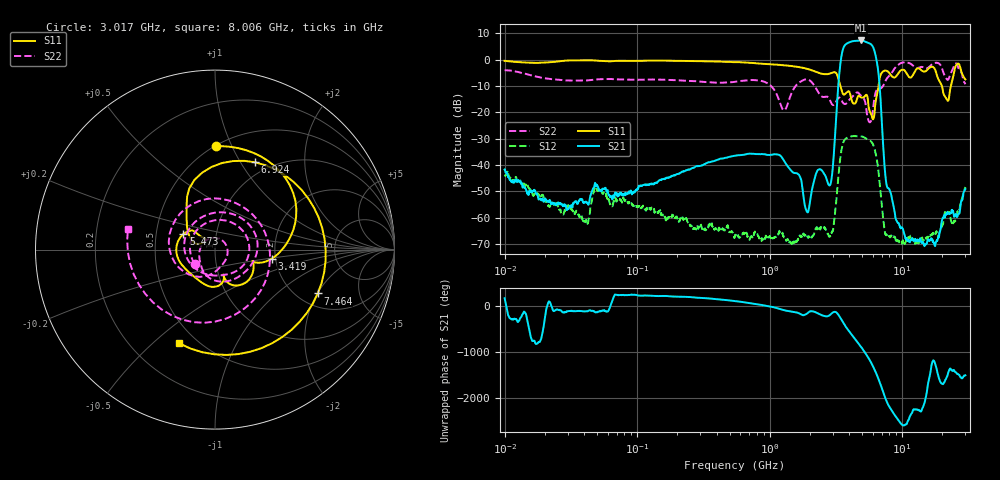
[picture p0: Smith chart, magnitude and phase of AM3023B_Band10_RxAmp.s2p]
# Hz S DB R 50.0
!freq dBS11 angS11 dBS21 angS21 dBS12 angS12 dBS22 angS22
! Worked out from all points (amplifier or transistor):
!   1601 points, 10 MHz to 30 GHz, reference 50 ohm
!   highest |S21| = 7.3 dB at 4.903 GHz (marker M1)
!   |S21| within 3 dB of that: 3.593 GHz to 6.089 GHz (2.496 GHz wide, 51.6 % of centre)
!   unconditionally stable (mu >= 1): start of sweep to end of sweep
!   at 37.85 MHz: K = 7082.18, MAG = -38.6 dB, |S12| = -58.9 dB
!   at 547.7 MHz: K = 11901.95, MAG = -28.6 dB, |S12| = -66.7 dB
!   at 30 GHz: K = 26834.51, MAG = -47.7 dB, |S12| = -48.3 dB
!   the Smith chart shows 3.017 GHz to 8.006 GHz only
!   S11 on the Smith chart (normalised r, x): 3.017 GHz: 0.51, +0.87; 3.419 GHz: 1.91, -0.21; 5.473 GHz: 0.69, +0.13; 6.924 GHz: 0.85, +1.16; 7.464 GHz: 2.53, -2.02; 8.006 GHz: 0.40, -0.61
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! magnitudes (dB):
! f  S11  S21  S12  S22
! 10 MHz  -0.4  -41.7  -44.3  -4.0
! 38.04 MHz  -0.2  -53.2  -59.2  -7.9
! 49.35 MHz  -0.3  -47.4  -48.7  -7.5
! 144.7 MHz  -0.3  -46.0  -58.0  -7.5
! 547.7 MHz  -0.9  -36.4  -66.7  -8.4
! 1.282 GHz  -2.1  -38.3  -67.4  -19.2
! 1.904 GHz  -3.4  -57.5  -66.9  -7.4
! 2.084 GHz  -4.0  -49.4  -67.2  -8.6
! 3.017 GHz  -4.8  -39.1  -64.4  -17.2
! 3.419 GHz  -9.9  -1.4  -37.1  -14.6
! 4.903 GHz  -14.3  7.3  -29.1  -13.7
! 5.473 GHz  -14.1  6.5  -30.2  -21.7
! 6.328 GHz  -15.5  1.2  -35.9  -12.2
! 6.924 GHz  -5.4  -18.0  -52.6  -10.8
! 7.464 GHz  -4.1  -43.8  -66.3  -8.2
! 7.926 GHz  -4.8  -48.9  -67.1  -6.3
! 8.006 GHz  -5.0  -49.2  -67.2  -6.0
! 10.86 GHz  -5.3  -68.4  -67.7  -1.0
! 14.81 GHz  -4.5  -70.3  -67.2  -3.1
! 21.67 GHz  -14.9  -58.6  -57.7  -7.3
! 25.95 GHz  -1.7  -59.5  -58.6  -1.6
! 30 GHz  -7.5  -49.1  -48.3  -9.3
